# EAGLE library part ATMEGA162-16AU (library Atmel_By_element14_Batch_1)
8-bit Microcontroller
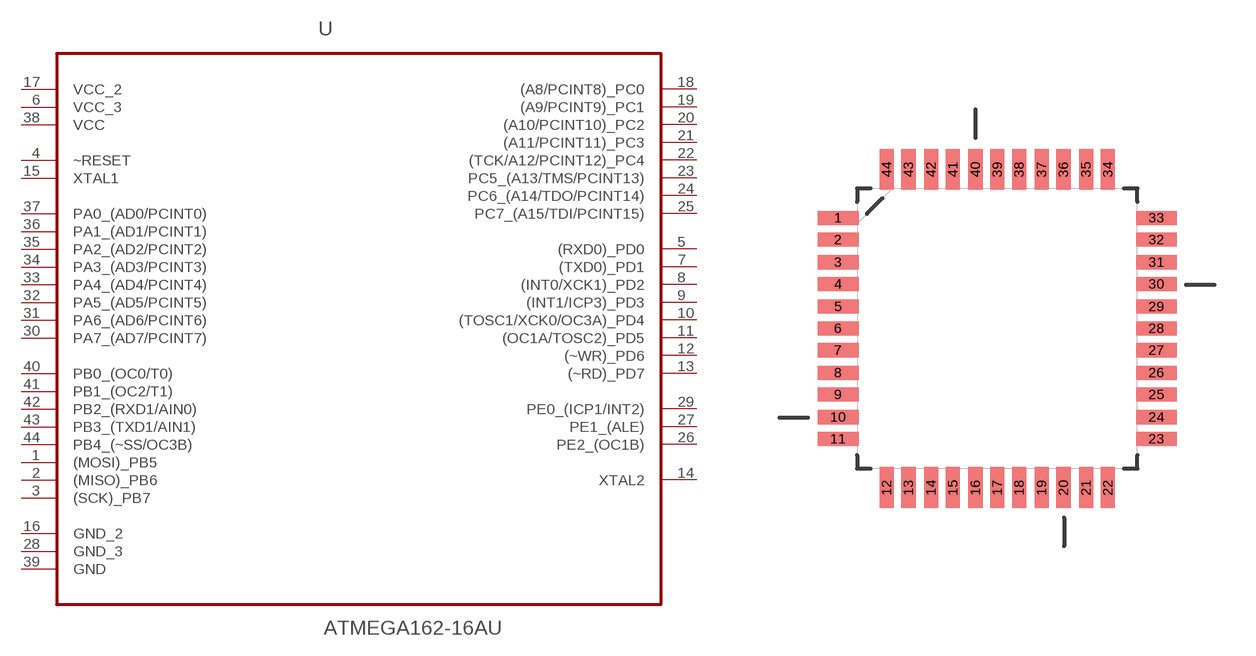
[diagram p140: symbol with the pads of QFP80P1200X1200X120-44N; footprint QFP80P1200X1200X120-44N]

Designator prefix U

## ATMEGA162-16AU (DESCRIPTION: 8-bit Microcontroller; MPN: ATMEGA162-16AU; OC_FARNELL: 9171150; OC_NEWARK: 96K6516; PACKAGE: QFP-44; SUPPLIER: Atmel)  [QFP80P1200X1200X120-44N]
1  (MOSI)_PB5
2  (MISO)_PB6
3  (SCK)_PB7
4  ~RESET  in
5  (RXD0)_PD0
6  VCC_3  pwr
7  (TXD0)_PD1
8  (INT0/XCK1)_PD2
9  (INT1/ICP3)_PD3
10  (TOSC1/XCK0/OC3A)_PD4
11  (OC1A/TOSC2)_PD5
12  (~WR)_PD6
13  (~RD)_PD7
14  XTAL2  out
15  XTAL1  in
16  GND_2  pas
17  VCC_2  pwr
18  (A8/PCINT8)_PC0
19  (A9/PCINT9)_PC1
20  (A10/PCINT10)_PC2
21  (A11/PCINT11)_PC3
22  (TCK/A12/PCINT12)_PC4
23  PC5_(A13/TMS/PCINT13)
24  PC6_(A14/TDO/PCINT14)
25  PC7_(A15/TDI/PCINT15)
26  PE2_(OC1B)
27  PE1_(ALE)
28  GND_3  pas
29  PE0_(ICP1/INT2)
30  PA7_(AD7/PCINT7)
31  PA6_(AD6/PCINT6)
32  PA5_(AD5/PCINT5)
33  PA4_(AD4/PCINT4)
34  PA3_(AD3/PCINT3)
35  PA2_(AD2/PCINT2)
36  PA1_(AD1/PCINT1)
37  PA0_(AD0/PCINT0)
38  VCC  pwr
39  GND  pas
40  PB0_(OC0/T0)
41  PB1_(OC2/T1)
42  PB2_(RXD1/AIN0)
43  PB3_(TXD1/AIN1)
44  PB4_(~SS/OC3B)

## Footprint QFP80P1200X1200X120-44N (pad centres in mm)
smd 1.473 x 0.508: 1 -5.74,3.988; 2 -5.74,3.2; 3 -5.74,2.388; 4 -5.74,1.6; 5 -5.74,0.787; 6 -5.74,0; 7 -5.74,-0.787; 8 -5.74,-1.6; 9 -5.74,-2.388; 10 -5.74,-3.2; 11 -5.74,-3.988; 23 5.74,-3.988; 24 5.74,-3.2; 25 5.74,-2.388; 26 5.74,-1.6; 27 5.74,-0.787; 28 5.74,0; 29 5.74,0.787; 30 5.74,1.6; 31 5.74,2.388; 32 5.74,3.2; 33 5.74,3.988
smd 0.508 x 1.473: 12 -3.988,-5.74; 13 -3.2,-5.74; 14 -2.388,-5.74; 15 -1.6,-5.74; 16 -0.787,-5.74; 17 0,-5.74; 18 0.787,-5.74; 19 1.6,-5.74; 20 2.388,-5.74; 21 3.2,-5.74; 22 3.988,-5.74; 34 3.988,5.74; 35 3.2,5.74; 36 2.388,5.74; 37 1.6,5.74; 38 0.787,5.74; 39 0,5.74; 40 -0.787,5.74; 41 -1.6,5.74; 42 -2.388,5.74; 43 -3.2,5.74; 44 -3.988,5.74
